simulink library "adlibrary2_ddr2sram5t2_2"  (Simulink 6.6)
undefined symbols (not defined in the file or in its folder): Bit, Location, Lower, Width
libraries: xbsIndex_r4 x20, adlibrary2_ddr2sram5t2_2 x1

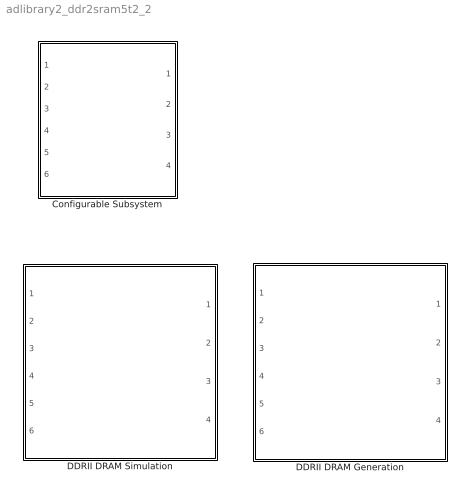
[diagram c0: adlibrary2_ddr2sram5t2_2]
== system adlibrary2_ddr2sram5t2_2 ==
  Configurable Subsystem : Subsystem  BlockChoice=DDRII DRAM Generation
  DDRII DRAM Generation : Subsystem
  DDRII DRAM Simulation : Subsystem

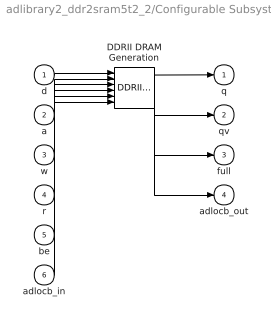
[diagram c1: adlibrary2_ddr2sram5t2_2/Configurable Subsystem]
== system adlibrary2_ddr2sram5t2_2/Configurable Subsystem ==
  d : Inport
  a : Inport  Port=2
  w : Inport  Port=3
  r : Inport  Port=4
  be : Inport  Port=5
  adlocb_in : Inport  Port=6
  DDRII DRAM Generation : adlibrary2_ddr2sram5t2_2/DDRII DRAM Generation  SystemSampleTime=-1
  q : Outport
  qv : Outport  Port=2
  full : Outport  Port=3
  adlocb_out : Outport  Port=4
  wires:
  d/1 -> DDRII DRAM Generation/1
  a/1 -> DDRII DRAM Generation/2
  w/1 -> DDRII DRAM Generation/3
  r/1 -> DDRII DRAM Generation/4
  be/1 -> DDRII DRAM Generation/5
  adlocb_in/1 -> DDRII DRAM Generation/6
  DDRII DRAM Generation/1 -> q/1
  DDRII DRAM Generation/2 -> qv/1
  DDRII DRAM Generation/3 -> full/1
  DDRII DRAM Generation/4 -> adlocb_out/1

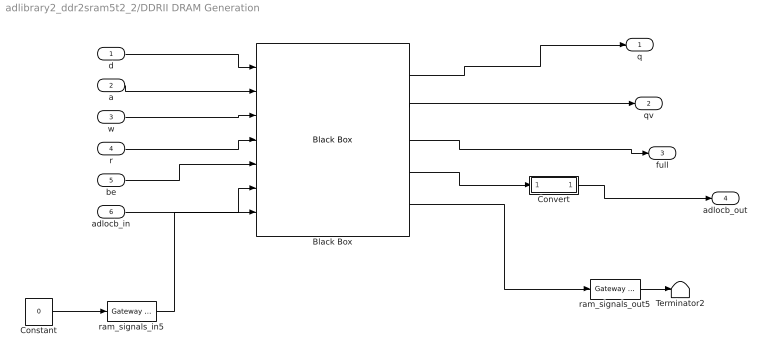
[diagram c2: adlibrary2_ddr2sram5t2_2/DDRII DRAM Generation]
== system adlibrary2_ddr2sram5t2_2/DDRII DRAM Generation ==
  d : Inport
  a : Inport  Port=2
  w : Inport  Port=3
  r : Inport  Port=4
  be : Inport  Port=5
  adlocb_in : Inport  Port=6
  Black Box : xbsIndex_r4/Black Box  init_code=ddr2sram_v5_config5  sim_method=Inactive  block_type=blackbox2
  Constant : Constant  Value=0
  Convert : Subsystem
  Terminator2 : Terminator
  ram_signals_in5 : xbsIndex_r4/Gateway In  arith_type=Unsigned  n_bits=69  bin_pt=0  quantization="Round  (unbiased: +/- Inf)"  overflow=Saturate  period=ad_get_simulink_period  dbl_ovrd=off  timing_constraint=None  locs_specified=off  LOCs={}  block_type=gatewayin
  ram_signals_out5 : xbsIndex_r4/Gateway Out  hdl_port=on  timing_constraint=None  locs_specified=off  LOCs={}  block_type=gatewayout
  q : Outport
  qv : Outport  Port=2
  full : Outport  Port=3
  adlocb_out : Outport  Port=4
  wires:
  ram_signals_out5/1 -> Terminator2/1
  Constant/1 -> ram_signals_in5/1
  d/1 -> Black Box/1
  a/1 -> Black Box/2
  w/1 -> Black Box/3
  r/1 -> Black Box/4
  be/1 -> Black Box/5
  adlocb_in/1 -> Black Box/6
  Black Box/1 -> q/1
  Black Box/2 -> qv/1
  Black Box/3 -> full/1
  Black Box/4 -> Convert/1(in0)
  Convert/1(out0) -> adlocb_out/1
  ram_signals_in5/1 -> Black Box/7
  Black Box/5 -> ram_signals_out5/1

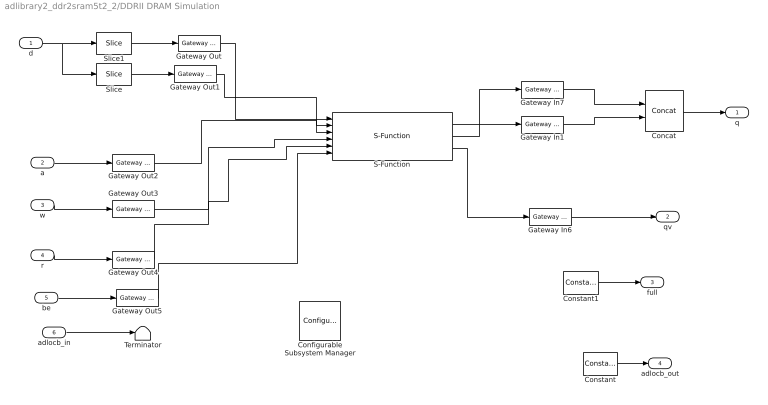
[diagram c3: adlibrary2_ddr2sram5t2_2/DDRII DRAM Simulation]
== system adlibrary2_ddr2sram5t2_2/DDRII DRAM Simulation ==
  d : Inport
  a : Inport  Port=2
  w : Inport  Port=3
  r : Inport  Port=4
  be : Inport  Port=5
  adlocb_in : Inport  Port=6
  Concat : xbsIndex_r4/Concat  num_inputs=2  dbl_ovrd=off  block_type=concat
  Configurable Subsystem Manager : xbsIndex_r4/Configurable Subsystem Manager  Tag=xcfgMgr  block_type=configsubsys
  Constant : xbsIndex_r4/Constant  arith_type=Signed (2's comp)  const=0  n_bits=66  bin_pt=0  explicit_period=on  period=ad_get_simulink_period  equ=P=C  opselect=C  inp2=PCIN>>17  opr=+  inp1=P  carry=CIN  dbl_ovrd=off  block_type=constant
  Constant1 : xbsIndex_r4/Constant  arith_type=Boolean  const=0  n_bits=66  bin_pt=0  explicit_period=on  period=ad_get_simulink_period  equ=P=C  opselect=C  inp2=PCIN>>17  opr=+  inp1=P  carry=CIN  dbl_ovrd=off  block_type=constant
  Gateway In1 : xbsIndex_r4/Gateway In  arith_type=Unsigned  n_bits=32  bin_pt=0  quantization="Round  (unbiased: +/- Inf)"  overflow=Saturate  period=ad_get_simulink_period  dbl_ovrd=on  timing_constraint=None  locs_specified=off  LOCs={}  block_type=gatewayin
  Gateway In6 : xbsIndex_r4/Gateway In  arith_type=Boolean  n_bits=1  bin_pt=0  quantization="Round  (unbiased: +/- Inf)"  overflow=Saturate  period=ad_get_simulink_period  dbl_ovrd=on  timing_constraint=None  locs_specified=off  LOCs={}  block_type=gatewayin
  Gateway In7 : xbsIndex_r4/Gateway In  arith_type=Unsigned  n_bits=32  bin_pt=0  quantization="Round  (unbiased: +/- Inf)"  overflow=Saturate  period=ad_get_simulink_period  dbl_ovrd=on  timing_constraint=None  locs_specified=off  LOCs={}  block_type=gatewayin
  Gateway Out{,1..5} (6 alike) : xbsIndex_r4/Gateway Out  hdl_port=off  timing_constraint=None  locs_specified=off  LOCs={}  block_type=gatewayout
  S-Function : S-Function  FunctionName=ddr2dram  Parameters=5
  Slice : xbsIndex_r4/Slice  nbits=32  boolean_output=off  mode=Lower Bit Location + Width  bit1=0  base1=MSB of Input  bit0=0  base0=LSB of Input  dbl_ovrd=off  block_type=slice
  Slice1 : xbsIndex_r4/Slice  nbits=32  boolean_output=off  mode=Lower Bit Location + Width  bit1=0  base1=MSB of Input  bit0=32  base0=LSB of Input  dbl_ovrd=off  block_type=slice
  Terminator : Terminator
  q : Outport
  qv : Outport  Port=2
  full : Outport  Port=3
  adlocb_out : Outport  Port=4
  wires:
  Concat/1 -> q/1
  d/1 -> Slice1/1, Slice/1
  Slice/1 -> Gateway Out1/1
  Slice1/1 -> Gateway Out/1
  Gateway Out5/1 -> S-Function/6
  be/1 -> Gateway Out5/1
  S-Function/3 -> Gateway In6/1
  Gateway In6/1 -> qv/1
  S-Function/2 -> Gateway In1/1
  Gateway Out4/1 -> S-Function/5
  r/1 -> Gateway Out4/1
  Gateway Out3/1 -> S-Function/4
  Gateway Out2/1 -> S-Function/3
  Gateway Out1/1 -> S-Function/2
  Gateway Out/1 -> S-Function/1
  S-Function/1 -> Gateway In7/1
  w/1 -> Gateway Out3/1
  a/1 -> Gateway Out2/1
  Constant/1 -> adlocb_out/1
  adlocb_in/1 -> Terminator/1
  Constant1/1 -> full/1
  Gateway In1/1 -> Concat/2
  Gateway In7/1 -> Concat/1

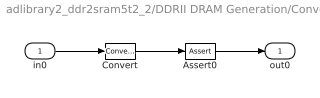
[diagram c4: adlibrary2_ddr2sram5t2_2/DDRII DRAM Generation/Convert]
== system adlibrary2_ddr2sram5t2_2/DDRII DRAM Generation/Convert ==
  in0 : Inport
  Assert0 : xbsIndex_r4/Assert  assert_type=off  type_source=Explicitly  arith_type="Signed  (2's comp)"  n_bits=16  bin_pt=14  assert_rate=on  rate_source=Explicitly  period=ad_get_simulink_period  output_port=on  block_type=assert
  Convert : xbsIndex_r4/Convert  arith_type=Unsigned  n_bits=66  bin_pt=0  quantization=Truncate  overflow=Wrap  latency=0  dbl_ovrd=off  pipeline=off  block_type=convert
  out0 : Outport
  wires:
  in0/1 -> Convert/1
  Convert/1 -> Assert0/1
  Assert0/1 -> out0/1
